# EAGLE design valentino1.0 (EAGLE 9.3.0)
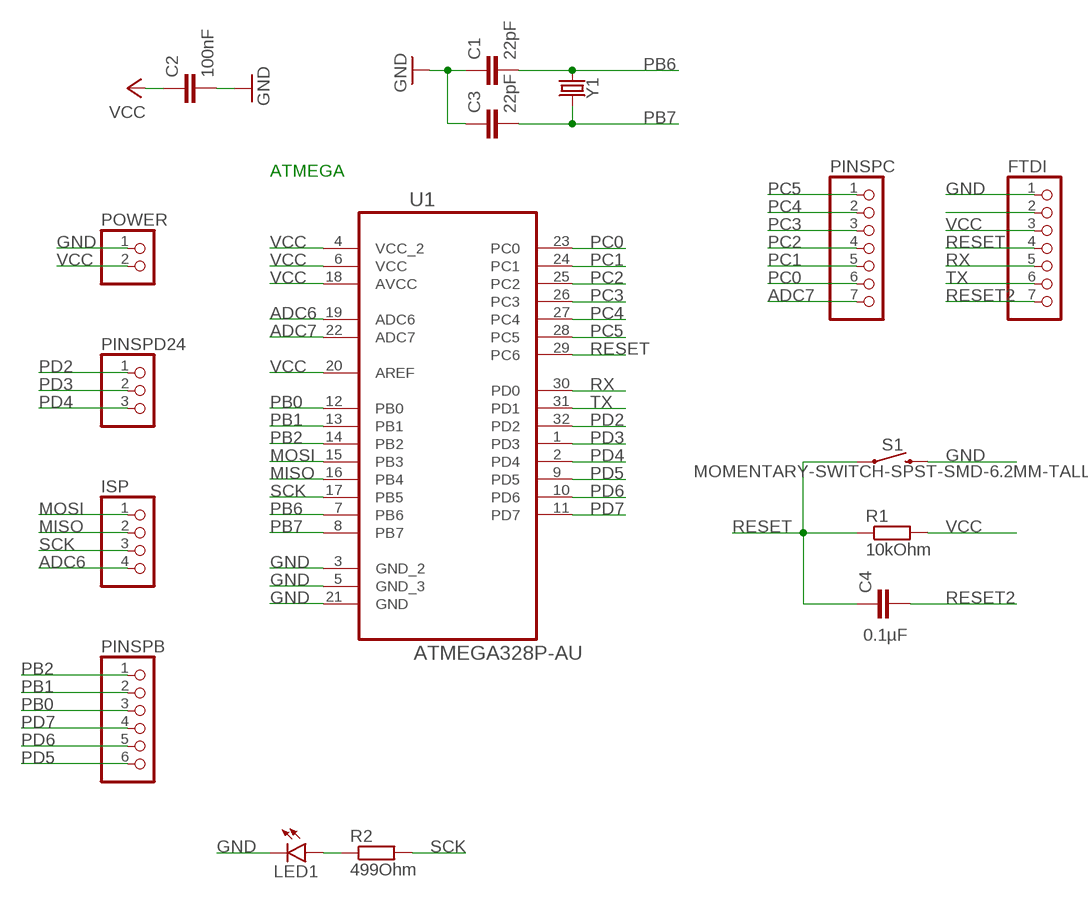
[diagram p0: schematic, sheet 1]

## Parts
C1  22pF  C-EUC1206  [C1206]
C2  100nF  C-EUC1206  [C1206]
C3  22pF  C-EUC1206  [C1206]
C4  0.1µF  C-EUC1206  [C1206]
FTDI  PINHD-1X7  [1X07]
ISP  PINHD-1X4  [1X04]
LED1  LEDSML1206  [SML1206]
PINSPB  PINHD-1X6  [1X06]
PINSPC  PINHD-1X7  [1X07]
PINSPD24  PINHD-1X3  [1X03]
POWER  PINHD-1X2  [1X02]
R1  10kOhm  R-EU_R1206  [R1206]
R2  499Ohm  R-EU_R1206  [R1206]
S1  MOMENTARY-SWITCH-SPST-SMD-6.2MM-TALL  [TACTILE_SWITCH_SMD_6.2MM_TALL]
U1  ATMEGA328P-AU  [QFP80P900X900X120-32N]
Y1  CRYSTALSMD-HC49UP  [HC49UP]

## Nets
ADC6: ISP.4 U1.19(ADC6)
ADC7: PINSPC.7 U1.22(ADC7)
GND: C1.1 C2.2 C3.1 FTDI.1 LED1.C POWER.1 S1.B2 U1.3(GND_2) U1.5(GND_3) U1.21(GND)
MISO: ISP.2 U1.16(PB4)
MOSI: ISP.1 U1.15(PB3)
N$2: LED1.A R2.1
N$19: FTDI.2
PB0: PINSPB.3 U1.12(PB0)
PB1: PINSPB.2 U1.13(PB1)
PB2: PINSPB.1 U1.14(PB2)
PB6: C1.2 U1.7(PB6) Y1.1
PB7: C3.2 U1.8(PB7) Y1.2
PC0: PINSPC.6 U1.23(PC0)
PC1: PINSPC.5 U1.24(PC1)
PC2: PINSPC.4 U1.25(PC2)
PC3: PINSPC.3 U1.26(PC3)
PC4: PINSPC.2 U1.27(PC4)
PC5: PINSPC.1 U1.28(PC5)
PD2: PINSPD24.1 U1.32(PD2)
PD3: PINSPD24.2 U1.1(PD3)
PD4: PINSPD24.3 U1.2(PD4)
PD5: PINSPB.6 U1.9(PD5)
PD6: PINSPB.5 U1.10(PD6)
PD7: PINSPB.4 U1.11(PD7)
RESET: C4.1 FTDI.4 R1.1 S1.A2 U1.29(PC6)
RESET2: C4.2 FTDI.7
RX: FTDI.5 U1.30(PD0)
SCK: ISP.3 R2.2 U1.17(PB5)
TX: FTDI.6 U1.31(PD1)
VCC: C2.1 FTDI.3 POWER.2 R1.2 U1.4(VCC_2) U1.6(VCC) U1.18(AVCC) U1.20(AREF)

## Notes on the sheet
- ATMEGA

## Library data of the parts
C1-C4 = rcl:C-EU: CAPACITOR, European symbol; SPICEPREFIX: C
FTDI PINSPC = pinhead:PINHD-1X7: PIN HEADER
ISP = pinhead:PINHD-1X4: PIN HEADER
LED1 = led:LED: LED
PINSPB = pinhead:PINHD-1X6: PIN HEADER
PINSPD24 = pinhead:PINHD-1X3: PIN HEADER
POWER = pinhead:PINHD-1X2: PIN HEADER
R1 R2 = rcl:R-EU_: RESISTOR, European symbol; SPICEPREFIX: R
S1 = SparkFun-Switches:MOMENTARY-SWITCH-SPST: Momentary Switch (Pushbutton) - SPST; PROD_ID: SWCH-11966; SF_SKU: COM-12992
U1 = Atmel_By_element14_Batch_1-00:ATMEGA328P-AU: 8-bit Microcontroller with In-System Programmable Flash; MPN: ATMEGA328P-AU; OC_FARNELL: 1715486; OC_NEWARK: 14R4631; PACKAGE: TQFP-32; SUPPLIER: Atmel
Y1 = SparkFun-Clocks:CRYSTAL: Crystals (Generic)

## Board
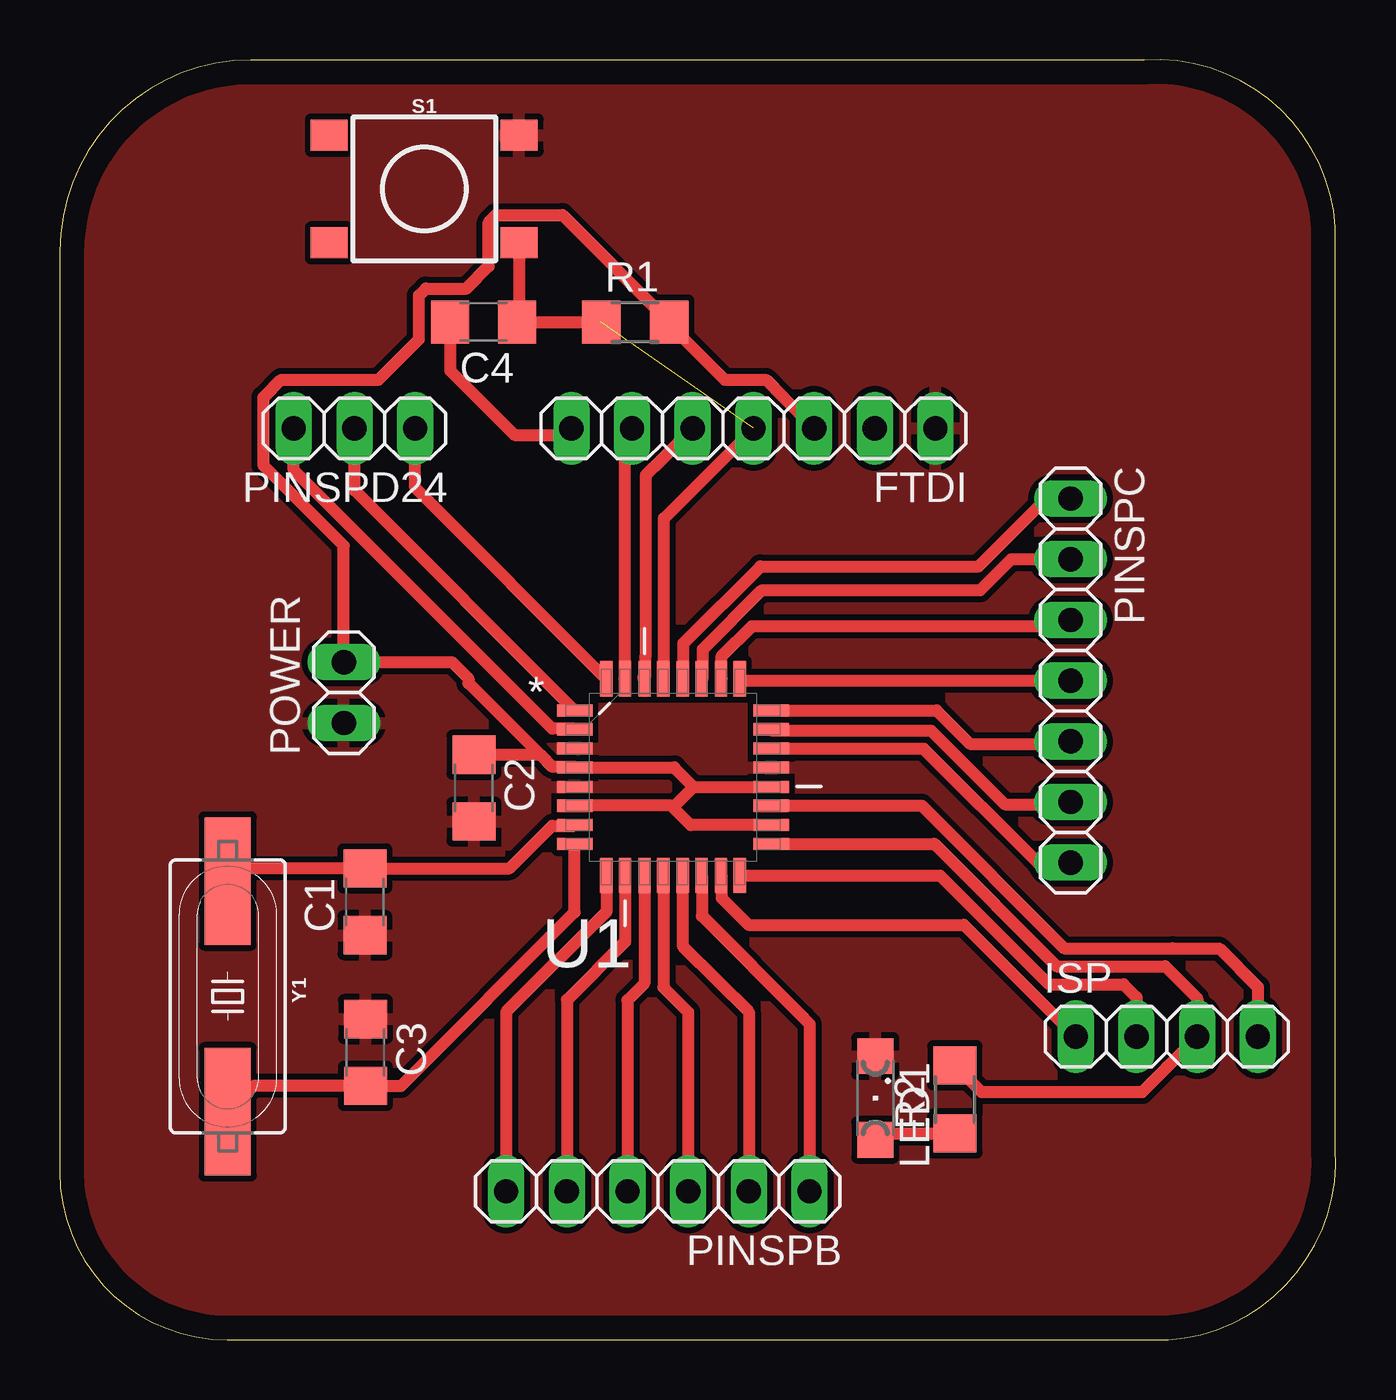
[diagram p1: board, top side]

Size 53.41 x 53.58 mm. Coordinates in mm from the lower left corner, seen from the top.
Outline: 0,45.56 0,7 arc90 7,0 46.4,0 arc90 53.4,8 53.4,46.56 arc90 45.4,53.56 8,53.56 arc90 0,45.56
Copper layers (1*16): Top 0.035mm / dielectric 1.5mm / Bottom 0.035mm
Design rules "default": minimum track width 0.2mm, minimum drill 0.35mm, track to track 0.25mm, track to pad 0.25mm, pad to pad 0.25mm, via to via 0.25mm, smd to smd 0.25mm, copper to edge 40mil, drill to drill 6mil, minimum pad ring 10mil, minimum via ring 8mil, stop-mask expansion 4mil, vias tented up to drill 0mil, thermal gap 10mil

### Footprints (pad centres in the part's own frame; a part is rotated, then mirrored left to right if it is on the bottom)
C1206 = smd 1.6 x 1.8: 1 -1.4,0; 2 1.4,0
1X07 = drill 1.016 long: 1 -7.62,0; 2 -5.08,0; 3 -2.54,0; 4 0,0; 5 2.54,0; 6 5.08,0; 7 7.62,0
1X04 = drill 1.016 long: 1 -3.81,0; 2 -1.27,0; 3 1.27,0; 4 3.81,0
SML1206 = smd 1.5 x 1.5: A 1.75,0; C -1.75,0
1X06 = drill 1.016 long: 1 -6.35,0; 2 -3.81,0; 3 -1.27,0; 4 1.27,0; 5 3.81,0; 6 6.35,0
1X03 = drill 1.016 long: 1 -2.54,0; 2 0,0; 3 2.54,0
1X02 = drill 1.016 long: 1 -1.27,0; 2 1.27,0
R1206 = smd 1.6 x 1.803: 1 -1.422,0; 2 1.422,0
TACTILE_SWITCH_SMD_6.2MM_TALL = smd 1.55 x 1.3: A1 -3.975,-2.25; A2 3.975,-2.25; B1 -3.975,2.25; B2 3.975,2.25
QFP80P900X900X120-32N = smd 1.473 x 0.508: 1 -4.115,2.794; 2 -4.115,2.007; 3 -4.115,1.194; 4 -4.115,0.406; 5 -4.115,-0.406; 6 -4.115,-1.194; 7 -4.115,-2.007; 8 -4.115,-2.794; 17 4.115,-2.794; 18 4.115,-2.007; 19 4.115,-1.194; 20 4.115,-0.406; 21 4.115,0.406; 22 4.115,1.194; 23 4.115,2.007; 24 4.115,2.794 | smd 0.508 x 1.473: 9 -2.794,-4.115; 10 -2.007,-4.115; 11 -1.194,-4.115; 12 -0.406,-4.115; 13 0.406,-4.115; 14 1.194,-4.115; 15 2.007,-4.115; 16 2.794,-4.115; 25 2.794,4.115; 26 2.007,4.115; 27 1.194,4.115; 28 0.406,4.115; 29 -0.406,4.115; 30 -1.194,4.115; 31 -2.007,4.115; 32 -2.794,4.115
HC49UP = smd 5.334 x 1.93: 1 -4.826,0; 2 4.826,0

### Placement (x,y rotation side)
C1  12.78,18.33 90 top
C2  17.34,23.09 270 top
C3  12.8,12.03 270 top
C4  17.74,42.6 180 top
FTDI  29.04,38.16 180 top
ISP  46.34,12.69 0 top
LED1  34.14,10.12 270 top
PINSPB  25.04,6.21 180 top
PINSPC  42.31,27.59 270 top
PINSPD24  12.34,38.16 180 top
POWER  11.89,27.09 90 top
R1  24.09,42.6 0 top
R2  37.47,10.06 90 top
S1  15.26,48.17 0 top
U1  25.67,23.55 0 top
Y1  7.03,14.38 270 top

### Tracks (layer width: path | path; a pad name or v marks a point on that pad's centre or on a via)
ADC6
  Top 0.508: U1.19 36.08,22.36 42.04,16.39 46.59,16.39 46.6,16.38 48.53,16.38 50.15,14.76 ISP.4
ADC7
  Top 0.508: U1.22 36.16,24.74 40.94,19.97 PINSPC.7
GND
  pour Top: -15.18,19.21 -15.18,39.31 arc-90 8.95,63.44 43.48,63.44 arc-90 66.09,40.81 66.09,17.71 arc-90 41.98,-6.4 10.45,-6.4 arc-90
MISO
  Top 0.508: U1.16 36.85,19.43 41.41,14.88 44.53,14.88 45.07,14.34 ISP.2
MOSI
  Top 0.508: U1.15 27.71,19.41 27.71,18.49 28.82,17.38 37.84,17.38 ISP.1
N$2
  Top 0.508: LED1.A 34.41,8.64 R2.1
PB0
  Top 0.508: U1.12 25.26,14.76 26.3,13.71 PINSPB.3
PB1
  Top 0.508: U1.13 26.08,16.5 27.57,15 27.57,14.99 28.84,13.71 PINSPB.2
PB2
  Top 0.508: U1.14 26.88,19.42 26.88,17.74 31.11,13.5 31.11,13.49 31.38,13.21 PINSPB.1
PB6
  Top 0.508: U1.7 21.53,21.51 20.61,21.51 18.83,19.73 C1.2 7.56,19.73 Y1.1
PB7
  Top 0.508: Y1.2 8.11,10.62 C3.2 14.28,10.62 21.55,17.9 U1.8
PC0
  Top 0.508: U1.23 29.84,25.5 36.48,25.5 39.57,22.41 42.21,22.41 PINSPC.6
PC1
  Top 0.508: U1.24 36.7,26.34 38.1,24.95 42.21,24.95 PINSPC.5
PC2
  Top 0.508: U1.25 28.54,27.59 PINSPC.4
PC3
  Top 0.508: U1.26 27.71,27.69 27.71,28.61 28.97,29.88 42.05,29.88 PINSPC.3
PC4
  Top 0.508: U1.27 26.92,27.72 26.92,28.89 29.4,31.38 38.53,31.38 39.83,32.67 PINSPC.2
PC5
  Top 0.508: U1.28 26.11,27.69 26.11,29.15 29.33,32.38 38.46,32.38 41.29,35.21 PINSPC.1
PD2
  Top 0.508: U1.32 14.88,35.67 PINSPD24.1
PD3
  Top 0.508: U1.1 12.34,35.56 PINSPD24.2
PD4
  Top 0.508: U1.2 21.53,25.59 20.61,25.59 9.8,36.4 PINSPD24.3
PD5
  Top 0.508: U1.9 22.88,17.91 18.69,13.71 PINSPB.6
PD6
  Top 0.508: U1.10 23.66,16.67 21.23,14.23 PINSPB.5
PD7
  Top 0.508: U1.11 24.48,14.93 23.77,14.21 PINSPB.4
RESET  (1 unrouted)
  Top 0.508: R1.1 C4.1 19.23,42.7 S1.A2 | U1.29 25.26,28.3 25.29,28.32 25.29,34.38 29.04,38.12 FTDI.4
RESET2
  Top 0.508: 16.84,42.1 C4.2 16.34,40.56 19.03,37.88 21.14,37.88 FTDI.7
RX
  Top 0.508: U1.30 24.42,27.72 24.51,27.8 24.51,28.61 24.53,28.64 24.53,36.18 25.22,36.87 25.22,36.88 FTDI.5
SCK
  Top 0.508: R2.2 38.58,10.38 45.31,10.38 46.34,11.4 46.34,11.41 ISP.3 47.61,14.29 46.27,15.63 41.73,15.63 36.6,20.76 U1.17
TX
  Top 0.508: 23.63,27.69 U1.31 23.66,37.86 FTDI.6 23.63,37.83
VCC
  Top 0.508: U1.18 26.41,21.54 25.59,22.36 | 25.59,22.36 U1.6 | 25.59,22.36 25.75,22.36 26.53,23.14 | 26.53,23.14 U1.20 | 26.53,23.14 25.72,23.96 U1.4 21.53,23.99 20.61,23.99 20.11,24.49 | 20.11,24.49 17.11,27.49 17.11,27.67 16.42,28.36 POWER.2 11.89,33.23 8.53,36.59 8.53,39.44 9.27,40.18 13.34,40.18 15.04,41.88 15.04,43.71 15.33,44 17.03,44 17.96,44.93 17.96,46.78 18.25,47.07 21.04,47.07 R1.2 25.55,42.57 25.55,42.47 27.83,40.18 29.56,40.18 30.3,39.44 30.3,39.43 FTDI.3 | C2.1 20.11,24.49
